| TEXAS INSTRUMENTS INCORPORATED
| Standard Linear and Logic Group
| IBIS Model of SN74LVC574A
| OCTAL EDGE-TRIGGERED D-TYPE FLIP-FLOPS WITH 3-STATE OUTPUTS
| This file contains package information for the following:
|  SSOP 20-pin (DB) package as [Component] LVC574A_DB
|  TVSOP 20-pin (DGV) package as [Component] LVC574A_DGV
|  SOIC 20-pin (DW) package as [Component] LVC574A_DW
|  PDIP 20-pin (N) package as [Component] LVC574A_N
|  SOP 20-pin (NS) package as [Component] LVC574A_NS
|  TSSOP 20-pin (PW) package as [Component] LVC574A_PW
|  QFN 20-pin (RGY) package as [Component] LVC574A_RGY
| This device can be powered at the following Vccs:
|  1.8 volt Vcc
|  2.5 volt Vcc
|  3.3 volt Vcc
| This file provides unique models under the [Model Selector] for each Vcc.
| For operation at a specific Vcc, select the appropriate model after each
| [Model Selector] keyword.
[IBIS Ver]   3.2
[Comment char]  |_char
[File Name]   sn74lvc574a.ibs
[File Rev]   1.2 | e_die
[Date]   September 4, 2003
[Source]   Data created from TI-SPICE simulations at TI-SLL.
[Notes]   The following is an IBIS list for the SN74LVC574A.
   Please contact sllibis@ti.com with questions and
   comments concerning SLL IBIS models.
   - C_comp values are taken at a different test condition than
   the Ci and Co in data sheet.
   - Power-clamp data has been deleted since there is no
   power-clamp diode in the device.
   - Due to the fact that the device is 5-V input/output
   tolerant, the pullup data has some non-monotonic warnings.
[Disclaimer] Property of Texas Instruments Incorporated. Unauthorized
   reproduction and/or distribution is strictly prohibited.
   This product is protected under copyright law.
   Created 2002, (C) Copyright 2002, Texas Instruments
   Incorporated, All Rights Reserved
   UNLESS THERE IS A SIGNED, WRITTEN AGREEMENT TO THE
   CONTRARY, TEXAS INSTRUMENTS (TI) IS PROVIDING THE IBIS
   MODELS  AND WITHOUT ANY WARRANTY, EXPRESSED OR
   IMPLIED. TI assumes no liability for:
   1) the accuracy of the IBIS models provided to your
   company;
   2) the proper functioning of these IBIS Models in your
   design or for any resulting applications; or
   3) infringement of patents, copyrights or intellectual
   property rights resulting from your use of these IBIS
   models.
   TI provides IBIS Models as a service to our customers.
   You and your company shall not distribute, sell or give
   these models to anyone else without prior written
   permission from TI.
   TI reserves the right to make changes to our products or
   to discontinue any semiconductor product or service
   without notice, and advises our customers to obtain the
   latest version of relevant information to verify, before
   placing orders, that the information being relied on is
   current.
   Please be aware that your receipt and use of the IBIS
   information provided shall serve as acceptance of these
   terms and conditions. If you do not accept these terms,
   you should return or destroy the IBIS models and any
   other accompanying information immediately.
| Component LVC574A_DB 20-pin SSOP
[Component]   LVC574A_DB
[Manufacturer]   Texas Instruments, Inc.
[Package]
|   typ   min   max
R_pkg   4.000e-02   3.500e-02   5.100e-02
L_pkg   3.495e-09   3.035e-09   4.314e-09
C_pkg   4.200e-13   3.460e-13   5.020e-13
[Pin]   signal_name   model_name   R_pin   L_pin   C_pin
1   NOE   LVC574A_OE   4.900e-02   4.310e-09   5.020e-13
2   1D   LVC574A_IN   4.800e-02   3.903e-09   4.870e-13
3   2D   LVC574A_IN   3.500e-02   3.189e-09   3.960e-13
4   3D   LVC574A_IN   3.500e-02   3.036e-09   3.470e-13
5   4D   LVC574A_IN   3.500e-02   3.035e-09   3.670e-13
6   5D   LVC574A_IN   3.500e-02   3.035e-09   3.670e-13
7   6D   LVC574A_IN   3.500e-02   3.036e-09   3.470e-13
8   7D   LVC574A_IN   3.500e-02   3.189e-09   3.970e-13
9   8D   LVC574A_IN   4.700e-02   3.899e-09   4.880e-13
10   GND   GND   5.100e-02   4.314e-09   5.000e-13
11   CLK   LVC574A_CLK   5.100e-02   4.314e-09   5.000e-13
12   8Q   LVC574A_OUT   4.700e-02   3.899e-09   4.880e-13
13   7Q   LVC574A_OUT   3.500e-02   3.189e-09   3.970e-13
14   6Q   LVC574A_OUT   3.500e-02   3.036e-09   3.460e-13
15   5Q   LVC574A_OUT   3.500e-02   3.035e-09   3.670e-13
16   4Q   LVC574A_OUT   3.500e-02   3.035e-09   3.670e-13
17   3Q   LVC574A_OUT   3.500e-02   3.036e-09   3.460e-13
18   2Q   LVC574A_OUT   3.500e-02   3.189e-09   3.970e-13
19   1Q   LVC574A_OUT   4.700e-02   3.899e-09   4.880e-13
20   VCC   POWER   5.100e-02   4.314e-09   5.020e-13
| Component LVC574A_DGV 20-pin TVSOP
[Component]   LVC574A_DGV
[Manufacturer]   Texas Instruments, Inc.
[Package]
|   typ   min   max
R_pkg   4.400e-02   3.800e-02   4.800e-02
L_pkg   2.561e-09   2.236e-09   2.961e-09
C_pkg   3.420e-13   2.640e-13   4.460e-13
[Pin]   signal_name   model_name   R_pin   L_pin   C_pin
1   NOE   LVC574A_OE   4.400e-02   2.935e-09   4.170e-13
2   1D   LVC574A_IN   4.200e-02   2.869e-09   4.460e-13
3   2D   LVC574A_IN   4.300e-02   2.399e-09   3.160e-13
4   3D   LVC574A_IN   4.400e-02   2.236e-09   2.650e-13
5   4D   LVC574A_IN   4.600e-02   2.278e-09   2.640e-13
6   5D   LVC574A_IN   4.500e-02   2.274e-09   2.640e-13
7   6D   LVC574A_IN   4.400e-02   2.285e-09   2.690e-13
8   7D   LVC574A_IN   4.300e-02   2.452e-09   3.200e-13
9   8D   LVC574A_IN   4.400e-02   2.900e-09   4.460e-13
10   GND   GND   4.400e-02   2.961e-09   4.180e-13
11   CLK   LVC574A_CLK   4.500e-02   2.954e-09   4.180e-13
12   8Q   LVC574A_OUT   4.200e-02   2.847e-09   4.430e-13
13   7Q   LVC574A_OUT   4.500e-02   2.453e-09   3.190e-13
14   6Q   LVC574A_OUT   4.500e-02   2.297e-09   2.690e-13
15   5Q   LVC574A_OUT   4.800e-02   2.334e-09   2.680e-13
16   4Q   LVC574A_OUT   4.800e-02   2.335e-09   2.670e-13
17   3Q   LVC574A_OUT   4.600e-02   2.299e-09   2.680e-13
18   2Q   LVC574A_OUT   4.600e-02   2.457e-09   3.200e-13
19   1Q   LVC574A_OUT   4.300e-02   2.848e-09   4.410e-13
20   VCC   POWER   3.800e-02   2.812e-09   4.080e-13
| Component LVC574A_DW 20-pin SOIC
[Component]   LVC574A_DW
[Manufacturer]   Texas Instruments, Inc.
[Package]
|   typ   min   max
R_pkg   3.800e-02   3.300e-02   4.500e-02
L_pkg   5.012e-09   4.110e-09   6.349e-09
C_pkg   7.170e-13   5.300e-13   8.680e-13
[Pin]   signal_name   model_name   R_pin   L_pin   C_pin
1   NOE   LVC574A_OE   4.200e-02   6.336e-09   8.650e-13
2   1D   LVC574A_IN   4.300e-02   5.542e-09   8.670e-13
3   2D   LVC574A_IN   3.400e-02   4.714e-09   7.320e-13
4   3D   LVC574A_IN   3.400e-02   4.377e-09   5.910e-13
5   4D   LVC574A_IN   3.600e-02   4.130e-09   5.330e-13
6   5D   LVC574A_IN   3.500e-02   4.111e-09   5.300e-13
7   6D   LVC574A_IN   3.400e-02   4.284e-09   5.830e-13
8   7D   LVC574A_IN   3.400e-02   4.634e-09   7.260e-13
9   8D   LVC574A_IN   4.000e-02   5.518e-09   8.650e-13
10   GND   GND   4.300e-02   6.349e-09   8.660e-13
11   CLK   LVC574A_CLK   4.100e-02   6.281e-09   8.610e-13
12   8Q   LVC574A_OUT   4.500e-02   5.561e-09   8.680e-13
13   7Q   LVC574A_OUT   3.300e-02   4.778e-09   7.420e-13
14   6Q   LVC574A_OUT   3.500e-02   4.414e-09   5.960e-13
15   5Q   LVC574A_OUT   3.500e-02   4.110e-09   5.330e-13
16   4Q   LVC574A_OUT   3.600e-02   4.130e-09   5.330e-13
17   3Q   LVC574A_OUT   3.400e-02   4.377e-09   5.910e-13
18   2Q   LVC574A_OUT   3.400e-02   4.714e-09   7.310e-13
19   1Q   LVC574A_OUT   4.300e-02   5.569e-09   8.680e-13
20   VCC   POWER   4.200e-02   6.308e-09   8.640e-13
| Component LVC574A_N 20-pin PDIP
[Component]   LVC574A_N
[Manufacturer]   Texas Instruments, Inc.
[Package]
|   typ   min   max
R_pkg   4.300e-02   3.800e-02   5.000e-02
L_pkg   7.384e-09   4.680e-09   1.032e-08
C_pkg   5.100e-13   2.310e-13   8.210e-13
[Pin]   signal_name   model_name   R_pin   L_pin   C_pin
1   NOE   LVC574A_OE   4.200e-02   9.427e-09   8.100e-13
2   1D   LVC574A_IN   4.600e-02   8.544e-09   4.560e-13
3   2D   LVC574A_IN   4.800e-02   7.163e-09   4.350e-13
4   3D   LVC574A_IN   4.000e-02   4.825e-09   2.610e-13
5   4D   LVC574A_IN   4.000e-02   5.284e-09   6.480e-13
6   5D   LVC574A_IN   4.000e-02   4.686e-09   2.320e-13
7   6D   LVC574A_IN   4.000e-02   6.359e-09   4.890e-13
8   7D   LVC574A_IN   3.800e-02   7.982e-09   4.750e-13
9   8D   LVC574A_IN   4.300e-02   9.403e-09   4.750e-13
10   GND   GND   5.000e-02   1.032e-08   8.050e-13
11   CLK   LVC574A_CLK   5.000e-02   1.028e-08   8.100e-13
12   8Q   LVC574A_OUT   4.300e-02   9.383e-09   4.770e-13
13   7Q   LVC574A_OUT   3.800e-02   7.978e-09   4.760e-13
14   6Q   LVC574A_OUT   4.000e-02   6.302e-09   4.920e-13
15   5Q   LVC574A_OUT   4.000e-02   4.680e-09   2.310e-13
16   4Q   LVC574A_OUT   4.000e-02   5.284e-09   6.480e-13
17   3Q   LVC574A_OUT   4.000e-02   4.822e-09   2.610e-13
18   2Q   LVC574A_OUT   4.700e-02   7.118e-09   4.390e-13
19   1Q   LVC574A_OUT   4.600e-02   8.492e-09   4.610e-13
20   VCC   POWER   4.300e-02   9.348e-09   8.210e-13
| Component LVC574A_NS 20-pin SOP
[Component]   LVC574A_NS
[Manufacturer]   Texas Instruments, Inc.
[Package]
|   typ   min   max
R_pkg   4.400e-02   2.900e-02   5.800e-02
L_pkg   3.666e-09   2.317e-09   5.115e-09
C_pkg   5.480e-13   3.160e-13   7.250e-13
[Pin]   signal_name   model_name   R_pin   L_pin   C_pin
1   NOE   LVC574A_OE   5.800e-02   5.115e-09   7.250e-13
2   1D   LVC574A_IN   5.300e-02   4.591e-09   7.240e-13
3   2D   LVC574A_IN   4.900e-02   3.754e-09   5.720e-13
4   3D   LVC574A_IN   2.900e-02   2.549e-09   3.880e-13
5   4D   LVC574A_IN   3.100e-02   2.317e-09   3.160e-13
6   5D   LVC574A_IN   3.100e-02   2.317e-09   3.160e-13
7   6D   LVC574A_IN   2.900e-02   2.556e-09   3.990e-13
8   7D   LVC574A_IN   4.900e-02   3.754e-09   5.790e-13
9   8D   LVC574A_IN   5.300e-02   4.591e-09   7.240e-13
10   GND   GND   5.800e-02   5.115e-09   7.250e-13
11   CLK   LVC574A_CLK   5.800e-02   5.115e-09   7.250e-13
12   8Q   LVC574A_OUT   5.300e-02   4.591e-09   7.240e-13
13   7Q   LVC574A_OUT   4.900e-02   3.754e-09   5.790e-13
14   6Q   LVC574A_OUT   2.900e-02   2.557e-09   3.990e-13
15   5Q   LVC574A_OUT   3.100e-02   2.317e-09   3.160e-13
16   4Q   LVC574A_OUT   3.100e-02   2.317e-09   3.160e-13
17   3Q   LVC574A_OUT   2.900e-02   2.557e-09   3.990e-13
18   2Q   LVC574A_OUT   4.900e-02   3.754e-09   5.790e-13
19   1Q   LVC574A_OUT   5.300e-02   4.591e-09   7.240e-13
20   VCC   POWER   5.800e-02   5.115e-09   7.250e-13
| Component LVC574A_PW 20-pin TSSOP
[Component]   LVC574A_PW
[Manufacturer]   Texas Instruments, Inc.
[Package]
|   typ   min   max
R_pkg   5.000e-02   4.200e-02   6.000e-02
L_pkg   2.802e-09   2.248e-09   3.553e-09
C_pkg   3.170e-13   2.020e-13   4.430e-13
[Pin]   signal_name   model_name   R_pin   L_pin   C_pin
1   NOE   LVC574A_OE   5.500e-02   3.461e-09   4.400e-13
2   1D   LVC574A_IN   5.500e-02   3.150e-09   4.010e-13
3   2D   LVC574A_IN   4.200e-02   2.619e-09   3.020e-13
4   3D   LVC574A_IN   4.500e-02   2.273e-09   2.020e-13
5   4D   LVC574A_IN   4.500e-02   2.248e-09   2.240e-13
6   5D   LVC574A_IN   4.500e-02   2.273e-09   2.260e-13
7   6D   LVC574A_IN   4.400e-02   2.323e-09   2.050e-13
8   7D   LVC574A_IN   4.600e-02   2.704e-09   3.070e-13
9   8D   LVC574A_IN   6.000e-02   3.265e-09   4.110e-13
10   GND   GND   5.700e-02   3.506e-09   4.360e-13
11   CLK   LVC574A_CLK   5.800e-02   3.553e-09   4.370e-13
12   8Q   LVC574A_OUT   5.800e-02   3.193e-09   4.050e-13
13   7Q   LVC574A_OUT   4.200e-02   2.704e-09   3.110e-13
14   6Q   LVC574A_OUT   4.600e-02   2.392e-09   2.100e-13
15   5Q   LVC574A_OUT   4.700e-02   2.334e-09   2.290e-13
16   4Q   LVC574A_OUT   4.700e-02   2.300e-09   2.270e-13
17   3Q   LVC574A_OUT   4.700e-02   2.349e-09   2.070e-13
18   2Q   LVC574A_OUT   4.500e-02   2.677e-09   3.060e-13
19   1Q   LVC574A_OUT   6.000e-02   3.235e-09   4.060e-13
20   VCC   POWER   5.600e-02   3.487e-09   4.430e-13
| Component LVC574A_RGY 20-pin QFN
[Component]   LVC574A_RGY
[Manufacturer]   Texas Instruments, Inc.
[Package]
|   typ   min   max
R_pkg   4.600e-02   3.500e-02   5.800e-02
L_pkg   1.131e-09   8.800e-10   1.396e-09
C_pkg   1.650e-13   1.420e-13   1.750e-13
[Pin]   signal_name   model_name   R_pin   L_pin   C_pin
1   NOE   LVC574A_OE   5.300e-02   1.289e-09   1.420e-13
2   1D   LVC574A_IN   5.800e-02   1.386e-09   1.720e-13
3   2D   LVC574A_IN   4.600e-02   1.111e-09   1.730e-13
4   3D   LVC574A_IN   3.900e-02   9.650e-10   1.610e-13
5   4D   LVC574A_IN   3.500e-02   8.810e-10   1.650e-13
6   5D   LVC574A_IN   3.500e-02   8.800e-10   1.650e-13
7   6D   LVC574A_IN   3.900e-02   9.610e-10   1.610e-13
8   7D   LVC574A_IN   4.500e-02   1.105e-09   1.720e-13
9   8D   LVC574A_IN   5.800e-02   1.386e-09   1.720e-13
10   GND   GND   5.600e-02   1.352e-09   1.590e-13
11   CLK   LVC574A_CLK   5.300e-02   1.287e-09   1.550e-13
12   8Q   LVC574A_OUT   5.800e-02   1.396e-09   1.720e-13
13   7Q   LVC574A_OUT   4.700e-02   1.129e-09   1.750e-13
14   6Q   LVC574A_OUT   4.000e-02   9.760e-10   1.640e-13
15   5Q   LVC574A_OUT   3.500e-02   8.840e-10   1.690e-13
16   4Q   LVC574A_OUT   3.500e-02   8.810e-10   1.680e-13
17   3Q   LVC574A_OUT   3.900e-02   9.670e-10   1.620e-13
18   2Q   LVC574A_OUT   4.600e-02   1.118e-09   1.740e-13
19   1Q   LVC574A_OUT   5.800e-02   1.396e-09   1.750e-13
20   VCC   POWER   5.200e-02   1.276e-09   1.440e-13
| Model LVC574A_CLK
[Model Selector]   LVC574A_CLK
LVC574A_CLK_18   1.8 volt Vcc
LVC574A_CLK_25   2.5 volt Vcc
LVC574A_CLK_33   3.3 volt Vcc
| Model LVC574A_OE
[Model Selector]   LVC574A_OE
LVC574A_OE_18   1.8 volt Vcc
LVC574A_OE_25   2.5 volt Vcc
LVC574A_OE_33   3.3 volt Vcc
| Model LVC574A_IN
[Model Selector]   LVC574A_IN
LVC574A_IN_18   1.8 volt Vcc
LVC574A_IN_25   2.5 volt Vcc
LVC574A_IN_33   3.3 volt Vcc
| Model LVC574A_OUT
[Model Selector]   LVC574A_OUT
LVC574A_OUT_18   1.8 volt Vcc
LVC574A_OUT_25   2.5 volt Vcc
LVC574A_OUT_33   3.3 volt Vcc
| Models and submodels in the file (12): LVC574A_CLK_18 (Input), LVC574A_CLK_25 (Input), LVC574A_CLK_33 (Input), LVC574A_OE_18 (Input), LVC574A_OE_25 (Input), LVC574A_OE_33 (Input), LVC574A_IN_18 (Input), LVC574A_IN_25 (Input), LVC574A_IN_33 (Input), LVC574A_OUT_18 (3-state), LVC574A_OUT_25 (3-state), LVC574A_OUT_33 (3-state)
